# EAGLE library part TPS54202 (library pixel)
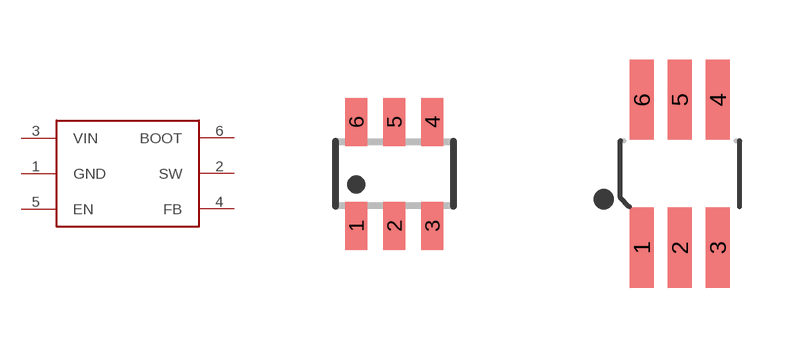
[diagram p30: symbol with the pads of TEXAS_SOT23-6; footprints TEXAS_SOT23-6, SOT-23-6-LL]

Designator prefix -

## TPS54202  [TEXAS_SOT23-6]
1  GND
2  SW
3  VIN
4  FB
5  EN
6  BOOT

## TPS54202LL  [SOT-23-6-LL]
Pads as for TEXAS_SOT23-6

## Footprint TEXAS_SOT23-6 (pad centres in mm)
SOT-23 - DBV 0.95 mm pitch
smd 0.55 x 1.2: 1 -0.95,-1.3; 2 0,-1.3; 3 0.95,-1.3; 4 0.95,1.3; 5 0,1.3; 6 -0.95,1.3

## Footprint SOT-23-6-LL (pad centres in mm)
smd 0.6 x 2: 1 -0.95,-1.85; 2 0,-1.85; 3 0.95,-1.85; 4 0.95,1.85; 5 0,1.85; 6 -0.95,1.85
